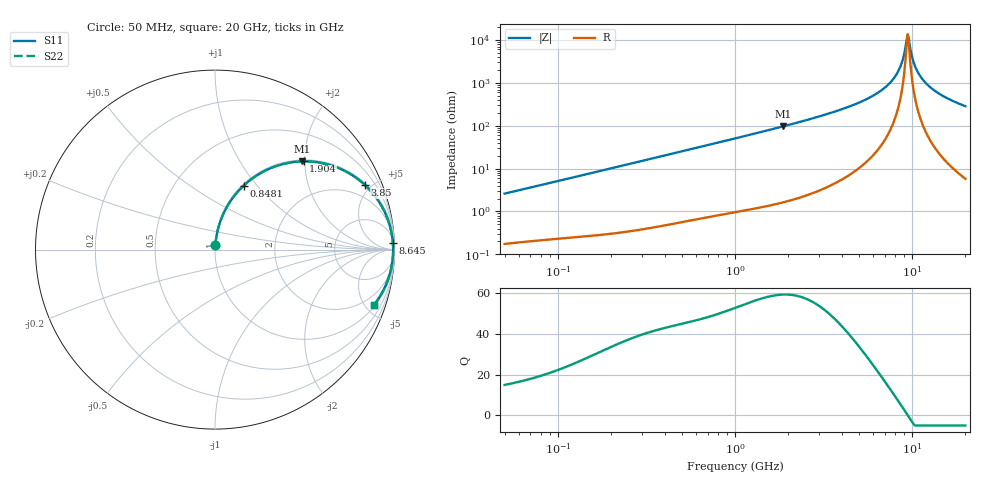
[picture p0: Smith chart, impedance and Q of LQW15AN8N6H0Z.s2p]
!Murata Part Number: LQW15AN8N6H0Z
!These Parameters are Measured in Series Mode Connection
!  o--[Z]--o
!Port1  Port2
!  o-------o
!Freq. Start=50[MHz] Stop=20[GHz], 401[Steps]
# Hz S RI R 50
!Freq.(Hz) S11(Real) S11(Imag) S21(Real) S21(Imag) S12(Real) S12(Imag) S22(Real) S22(Imag)
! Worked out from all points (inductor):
!   401 points, 50 MHz to 20 GHz, reference 50 ohm
!   read as one part in series: L = 8.24 nH near 51.52 MHz
!   highest Q = 59.2 at 1.876 GHz (marker M1), where L = 8.23 nH
!   self-resonance near 9.317 GHz
!   S11 on the Smith chart (normalised r, x): 50 MHz: 1.00, +0.05; 848.1 MHz: 1.02, +0.86; 1.904 GHz: 1.03, +1.97; 3.85 GHz: 1.10, +4.58; 8.645 GHz: 11, +50; 20 GHz: 1.12, -5.71
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5e7  0.00242 0.0259  0.9976 -0.0259  0.9976 -0.0259  0.00242 0.0259
1.364002e8  0.00735 0.0689  0.9926 -0.0689  0.9926 -0.0689  0.00735 0.0689
3.721004e8  0.0382 0.1802  0.9618 -0.1802  0.9618 -0.1802  0.0382 0.1802
8.480927e8  0.1595 0.3564  0.8405 -0.3564  0.8405 -0.3564  0.1595 0.3564
1e9  0.2077 0.3962  0.7923 -0.3962  0.7923 -0.3962  0.2077 0.3962
1.875929e9  0.4854 0.4914  0.5146 -0.4914  0.5146 -0.4914  0.4854 0.4914
1.904239e9  0.4933 0.4916  0.5067 -0.4916  0.5067 -0.4916  0.4933 0.4916
2.728004e9  0.6827 0.4565  0.3173 -0.4565  0.3173 -0.4565  0.6827 0.4565
3.850025e9  0.8344 0.3609  0.1656 -0.3609  0.1656 -0.3609  0.8344 0.3609
5.769027e9  0.947 0.2061  0.053 -0.2061  0.053 -0.2061  0.947 0.2061
7.442007e9  0.9821 0.1005  0.0179 -0.1005  0.0179 -0.1005  0.9821 0.1005
8.141811e9  0.9885 0.0628  0.0115 -0.0628  0.0115 -0.0628  0.9885 0.0628
8.644534e9  0.9911 0.0377  0.0089 -0.0377  0.0089 -0.0377  0.9911 0.0377
8.907419e9  0.9919 0.0251  0.00807 -0.0251  0.00807 -0.0251  0.9919 0.0251
9.178299e9  0.9924 0.0125  0.00757 -0.0125  0.00757 -0.0125  0.9924 0.0125
9.457416e9  0.9926 -8.05e-05  0.00738 8.05e-05  0.00738 8.05e-05  0.9926 -8.05e-05
9.600142e9  0.9926 -0.00638  0.00741 0.00638  0.00741 0.00638  0.9926 -0.00638
1.019291e10  0.9917 -0.0316  0.00833 0.0316  0.00833 0.0316  0.9917 -0.0316
1.050288e10  0.9907 -0.0441  0.00927 0.0441  0.00927 0.0441  0.9907 -0.0441
1.183995e10  0.9837 -0.0945  0.0163 0.0945  0.0163 0.0945  0.9837 -0.0945
1.460232e10  0.9583 -0.182  0.0417 0.182  0.0417 0.182  0.9583 -0.182
2e10  0.8858 -0.3081  0.1142 0.3081  0.1142 0.3081  0.8858 -0.3081
